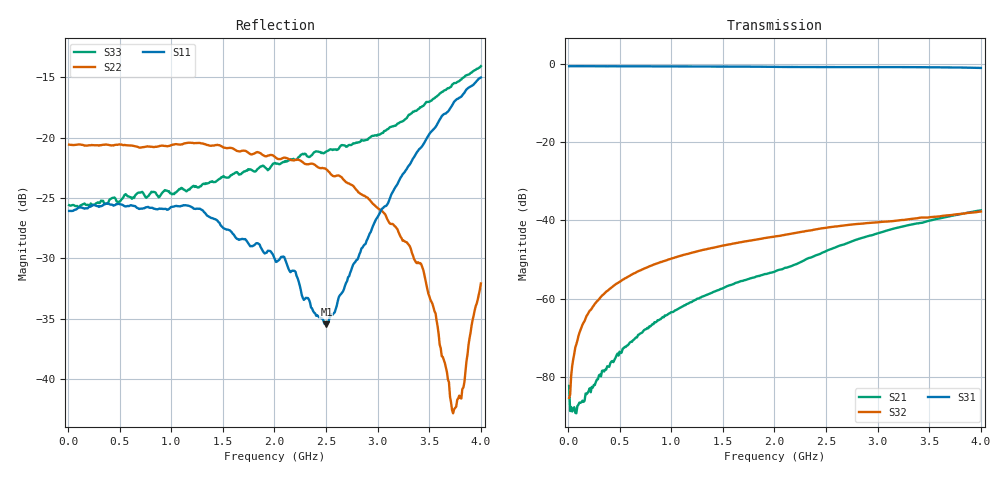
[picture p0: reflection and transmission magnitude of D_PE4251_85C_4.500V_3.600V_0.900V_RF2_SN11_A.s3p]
! Device ID: PE4251_SoldCshunt_081809
! Dir: c:\Test Bench Repositories\Bench_Software_CVI_Version_8\trunk\PSC 4Port_VNA Bench\datalog\4250\TEST\PE4251_SoldCshunt_081809\85C\4p500000\RF2
! Serial: 11
! Insertion: A
! Temp: 85C
! VDD: 4.500
! Control_Hi: 80.000
! Control_Lo: 20.000
! Logic State: RF2
! Port 1: RFC
! Port 2: RF1
! Port 3: RF2
! V1 = 0.90
! V2 = 0.90
! V3 = 0.90
! IDD: 5.831530e-05
! FILE NAME
! DATE 08/18/09  20:18
! CORRECTED  DATA
#  Hz  S  RI  R  50.00
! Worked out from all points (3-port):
!   401 points, 10 MHz to 4 GHz, reference 50 ohm
!   strongest paths, dB at 10 MHz, 1.008 GHz, 2.005 GHz, 3.002 GHz, 4 GHz:
!     S31: -0.6, -0.7, -0.8, -0.8, -1.0
!     S32: -85.3, -49.7, -44.1, -40.5, -37.7
!     S21: -82.3, -63.4, -53.0, -43.3, -37.4
!   lowest |S11| = -35.5 dB at 2.504 GHz (marker M1), VSWR 1.03, Z = 50.4 - j1.64 ohm
!   |S11| at or under -10 dB: start of sweep to end of sweep
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1e7  0.0497 -0.000469  -3.78e-05 -5.33e-05  0.9306 -0.00398
     7.7e-05 -1.18e-06  0.0935 -0.00081  3.98e-05 -3.52e-06
     0.9315 -0.0052  4.73e-05 2.65e-05  0.0525 0.000506
9.9775e7  0.0512 0.00055  2.24e-05 -3.82e-05  0.9308 -0.0363
          2.58e-05 -3.59e-05  0.0937 -0.00269  4.4e-05 0.000336
          0.9321 -0.0357  4.94e-05 0.000327  0.0514 -0.000402
1.8955e8  0.0509 0.000119  3.01e-06 -6.84e-05  0.9281 -0.0667
          6.66e-06 -6.24e-05  0.0926 -0.00472  6.75e-05 0.00063
          0.9294 -0.0665  6.18e-05 0.000628  0.0526 -0.000885
4.58875e8  0.0526 -0.00311  -0.000126 -0.000128  0.9151 -0.1593
           -0.000123 -0.000124  0.0926 -0.0116  0.000141 0.00151
           0.9165 -0.1592  0.00014 0.00152  0.0555 -0.00674
9.8755e8  0.0495 -0.0127  -0.00063 -0.000172  0.8648 -0.3302
          -0.000633 -0.000165  0.0889 -0.0256  0.000432 0.00319
          0.8661 -0.3301  0.000417 0.00318  0.0573 -0.0135
2.005e9  0.0304 -0.00729  -0.00221 -7.7e-05  0.6857 -0.6035
         -0.00223 -8.14e-05  0.0767 -0.0322  0.00104 0.00615
         0.6873 -0.6034  0.00104 0.00616  0.0686 -0.0383
2.50375e9  0.00444 -0.0162  -0.00406 -0.000395  0.5753 -0.7006
           -0.00406 -0.000398  0.0678 -0.0293  0.00139 0.00794
           0.5772 -0.7003  0.00139 0.00794  0.0504 -0.0717
3.42145e9  -0.0823 -0.0392  -0.0091 0.00192  0.3236 -0.845
           -0.00909 0.00192  0.0241 -0.0176  0.00203 0.0106
           0.3268 -0.8449  0.00202 0.0107  -0.0358 -0.1289
3.74065e9  -0.1355 -0.0386  -0.0111 0.00349  0.2123 -0.8713
           -0.0111 0.00346  -0.00105 -0.00741  0.0019 0.0117
           0.2144 -0.8706  0.00191 0.0117  -0.0923 -0.1408
4e9  -0.175 -0.0304  -0.0125 0.00506  0.1173 -0.8789
     -0.0125 0.00502  -0.0248 -0.00214  0.00198 0.0128
     0.1194 -0.8782  0.00196 0.0128  -0.1419 -0.1378
